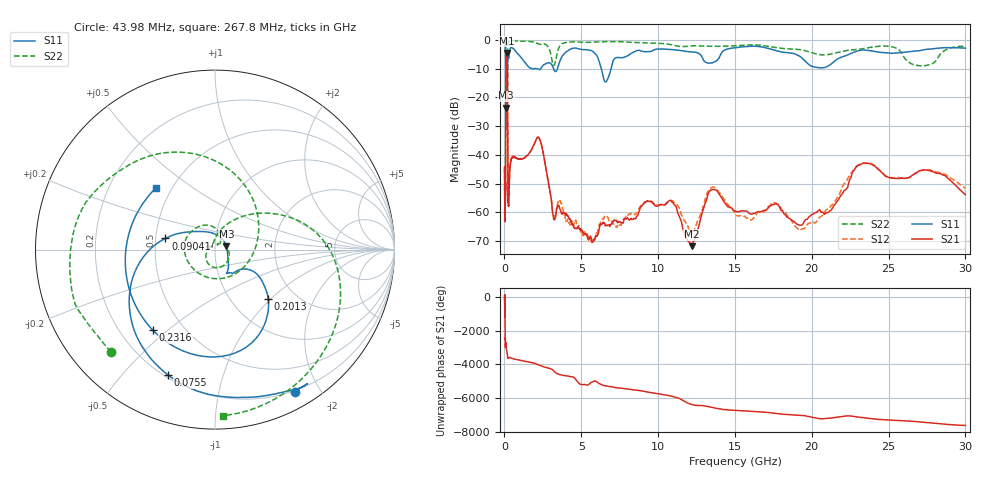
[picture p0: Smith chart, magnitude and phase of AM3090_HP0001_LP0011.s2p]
! Date/Time: Thu, Feb 28, 2019 1:54 PM
! Network Analyzer: Agilent Technologies E8364B Rev: A.07.50.67
! Sweep from 0.010 to 30.000 GHz, 1601 Points, Sweep Type: LOG
! Power Supply: 5.023 V, 0.002 A
# Hz S DB R 50
!freq MagS11 AngS11 MagS21 AngS21 MagS12 AngS12 MagS22 AngS22
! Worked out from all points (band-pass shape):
!   1601 points, 10 MHz to 30 GHz, reference 50 ohm
!   highest |S21| = -4.51 dB at 139 MHz (marker M1); lowest = -71.7 dB at 12.19 GHz (marker M2)
!   |S21| within 3 dB of the highest: 99.15 MHz to 187.9 MHz (88.72 MHz wide, 61.8 % of centre)
!   lowest |S11| = -23.6 dB at 98.44 MHz (marker M3), VSWR 1.14, Z = 56.7 + j2.19 ohm
!   |S11| at or under -10 dB: 2.137 GHz to 2.359 GHz (222.9 MHz wide, 9.92 % of centre); 3.201 GHz to 3.451 GHz (249.5 MHz wide, 7.5 % of centre); 6.308 GHz to 6.937 GHz (628.5 MHz wide, 9.49 % of centre)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
!   |S22| runs from -31.3 to -0.2 dB; largest |S21 - S12| = 0.011
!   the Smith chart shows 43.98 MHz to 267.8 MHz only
!   S11 on the Smith chart (normalised r, x): 43.98 MHz: 0.19, -1.70; 75.5 MHz: 0.21, -0.67; 90.41 MHz: 0.56, +0.08; 201.3 MHz: 1.46, -0.97; 231.6 MHz: 0.34, -0.44; 267.8 MHz: 0.41, +0.36
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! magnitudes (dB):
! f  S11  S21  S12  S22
! 10 MHz  -0.2  -46.2  -49.2  -0.5
! 38.04 MHz  -0.5  -59.7  -60.0  -1.4
! 43.98 MHz  -0.8  -58.2  -59.6  -1.8
! 75.5 MHz  -2.5  -44.8  -44.8  -4.8
! 90.41 MHz  -10.9  -14.7  -14.7  -15.7
! 98.44 MHz  -23.6  -7.8  -7.8  -15.3
! 139 MHz  -16.1  -4.5  -4.5  -24.2
! 144.7 MHz  -15.8  -4.5  -4.5  -21.7
! 179.4 MHz  -14.1  -6.1  -6.1  -31.3
! 201.3 MHz  -7.9  -14.5  -14.4  -11.3
! 231.6 MHz  -4.9  -55.6  -53.9  -1.6
! 267.8 MHz  -6.5  -57.9  -54.9  -0.7
! 550.5 MHz  -2.9  -40.6  -40.6  -0.3
! 2.084 GHz  -10.0  -34.4  -34.4  -1.0
! 3.236 GHz  -10.5  -62.5  -61.5  -8.8
! 7.926 GHz  -5.8  -62.3  -60.8  -0.7
! 10.76 GHz  -3.3  -55.8  -55.7  -1.5
! 12.19 GHz  -4.1  -71.7  -66.8  -2.0
! 13.61 GHz  -7.8  -52.1  -51.2  -2.2
! 19.51 GHz  -7.0  -63.2  -65.7  -3.6
! 23.36 GHz  -3.5  -42.8  -43.0  -3.0
! 30 GHz  -2.8  -53.8  -51.6  -2.2
